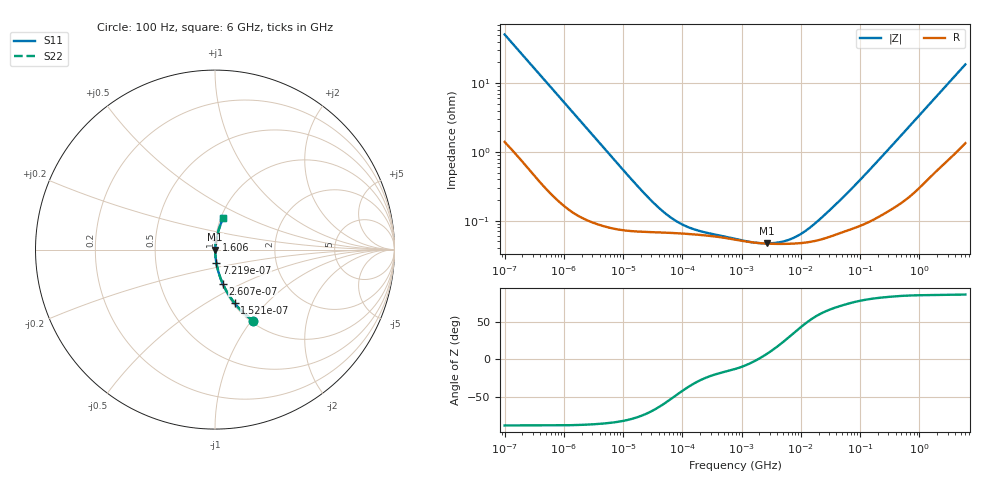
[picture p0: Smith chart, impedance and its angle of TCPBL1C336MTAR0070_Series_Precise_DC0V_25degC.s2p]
! TCPBL1C336MTAR0070 Polymer Tantalum Capacitor Sparameter Model
! Model Generated by Samsung Electro-Mechanics
! Samsung Sparameter Version 5.0
! Date : Oct-21-2025
! Products : Polymer Tantalum Capacitor
! Characteristics :
!  Nominal Capacitance = 33uF
!  Capacitance Tolerance = +/-20%
!  ESR = 70 mohm max at 100kHz
!  Rated Voltage = 16Vdc
!  Size = 1411(unit:inch), 3528(unit:mm)
!  Length = 3.50+/-0.20mm
!  Width = 2.80+/-0.20mm
!  Thickness = 1.10+/-0.10mm
!  Lineup = Conductive Polymer Type
!  Feature = PBL
!  Measurement Temperature : 25degC.
!  DC bias Value = 0V
!  Frequency : 100Hz ~ 6GHz
! External Node Assignments :
!  1  o---||---o  2
# MHz S RI R 50.0
! Freq.  Real(S11)  Im(S11)  Real(S12)  Im(S12)  Real(S21)  Im(S21)  Real(S22)  Im(S22)
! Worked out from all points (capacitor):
!   300 points, 100 Hz to 6 GHz, reference 50 ohm
!   read as one part in series: C = 31 uF near 106.2 Hz
!   lowest |Z| = 46.6 mohm at 2.645 MHz (marker M1)
!   series resonance near 1.922 MHz, so ESL is about 220 pH
!   S11 on the Smith chart (normalised r, x): 100 Hz: 1.03, -1.02; 152.1 Hz: 1.02, -0.68; 260.7 Hz: 1.01, -0.40; 721.9 Hz: 1.00, -0.15; 1.606 GHz: 1.01, +0.11; 6 GHz: 1.03, +0.37
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0.0001  0.2134 -0.3962  0.7866 0.3962  0.7866 0.3962  0.2134 -0.3962
0.0001520888  0.1095 -0.2986  0.8905 0.2986  0.8905 0.2986  0.1095 -0.2986
0.0002607487  0.0431 -0.1898  0.9569 0.1898  0.9569 0.1898  0.0431 -0.1898
0.0007218686  0.00738 -0.0724  0.9926 0.0724  0.9926 0.0724  0.00738 -0.0724
0.001998454  0.00181 -0.0266  0.9982 0.0266  0.9982 0.0266  0.00181 -0.0266
0.01626223  0.000707 -0.00334  0.9993 0.00334  0.9993 0.00334  0.000707 -0.00334
0.03993819  0.000676 -0.00138  0.9993 0.00138  0.9993 0.00138  0.000676 -0.00138
0.0726988  0.000659 -0.000788  0.9993 0.000788  0.9993 0.000788  0.000659 -0.000788
0.1246385  0.00064 -0.000488  0.9994 0.000488  0.9994 0.000488  0.00064 -0.000488
0.2268773  0.000613 -0.000302  0.9994 0.000302  0.9994 0.000302  0.000613 -0.000302
0.7981464  0.000526 -0.000121  0.9995 0.000121  0.9995 0.000121  0.000526 -0.000121
1.542536  0.000482 -3.38e-05  0.9995 3.38e-05  0.9995 3.38e-05  0.000482 -3.38e-05
2.644602  0.000463 5.39e-05  0.9995 -5.39e-05  0.9995 -5.39e-05  0.000463 5.39e-05
4.270427  0.000458 0.000151  0.9995 -0.000151  0.9995 -0.000151  0.000458 0.000151
6.895764  0.000461 0.000285  0.9995 -0.000285  0.9995 -0.000285  0.000461 0.000285
10.48768  0.000473 0.000453  0.9995 -0.000453  0.9995 -0.000453  0.000473 0.000453
15.95059  0.000499 0.000695  0.9995 -0.000695  0.9995 -0.000695  0.000499 0.000695
63.25518  0.000731 0.00249  0.9993 -0.00249  0.9993 -0.00249  0.000731 0.00249
318.7652  0.00154 0.0113  0.9985 -0.0113  0.9985 -0.0113  0.00154 0.0113
1606.371  0.00725 0.0527  0.9928 -0.0527  0.9928 -0.0527  0.00725 0.0527
3296.191  0.0187 0.1028  0.9813 -0.1028  0.9813 -0.1028  0.0187 0.1028
6000  0.0457 0.1762  0.9543 -0.1762  0.9543 -0.1762  0.0457 0.1762
